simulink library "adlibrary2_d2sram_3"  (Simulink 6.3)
undefined symbols (not defined in the file or in its folder): adlibrary2_zbt32_0, b9ac2330, Bit, Black, blackbox2, blue, Box1, d2sram_config, gcbh, Generation, Inactive, Location, Lower, SRAM, VER_STRING_GOES_HERE, white, Width, xlBlockLoadCallback, ZBT
libraries: xbsIndex_r4 x25, adlibrary2_d2sram_0 x1

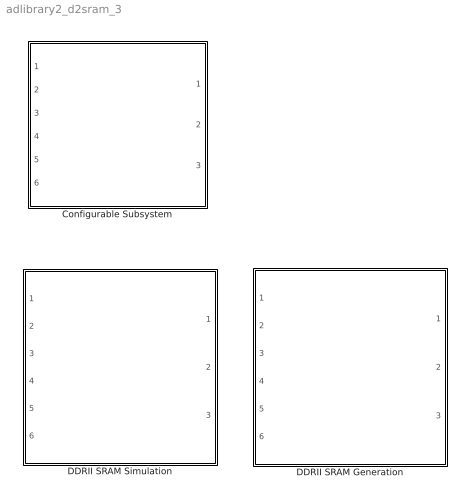
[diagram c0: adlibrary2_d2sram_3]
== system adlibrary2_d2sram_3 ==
  Configurable Subsystem : Subsystem  Tag=configX  BlockChoice=DDRII SRAM Simulation
  DDRII SRAM Generation : Subsystem
  DDRII SRAM Simulation : Subsystem

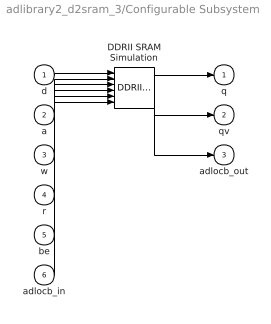
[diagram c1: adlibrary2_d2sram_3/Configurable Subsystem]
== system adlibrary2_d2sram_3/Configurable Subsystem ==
  d : Inport
  a : Inport  Port=2
  w : Inport  Port=3
  r : Inport  Port=4
  be : Inport  Port=5
  adlocb_in : Inport  Port=6
  DDRII SRAM Simulation : adlibrary2_d2sram_0/DDRII SRAM Simulation
  q : Outport
  qv : Outport  Port=2
  adlocb_out : Outport  Port=3
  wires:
  d/1 -> DDRII SRAM Simulation/1
  a/1 -> DDRII SRAM Simulation/2
  w/1 -> DDRII SRAM Simulation/3
  r/1 -> DDRII SRAM Simulation/4
  be/1 -> DDRII SRAM Simulation/5
  adlocb_in/1 -> DDRII SRAM Simulation/6
  DDRII SRAM Simulation/1 -> q/1
  DDRII SRAM Simulation/2 -> qv/1
  DDRII SRAM Simulation/3 -> adlocb_out/1

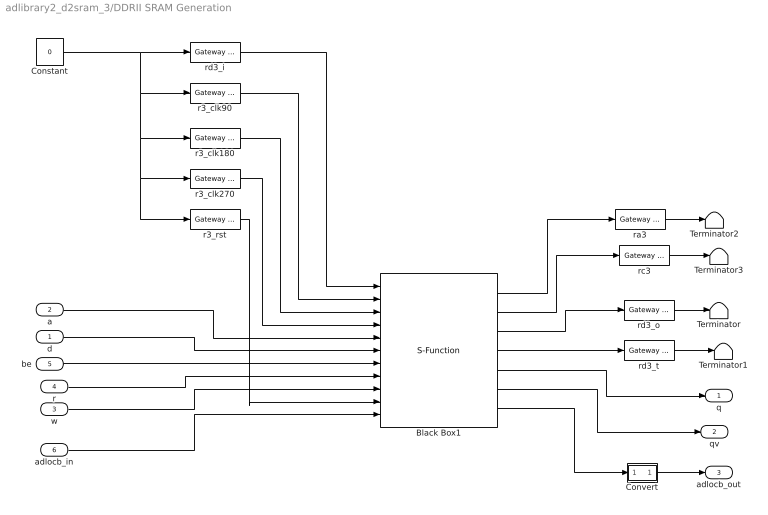
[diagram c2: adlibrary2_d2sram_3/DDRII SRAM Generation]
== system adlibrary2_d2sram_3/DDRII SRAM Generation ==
  d : Inport
  a : Inport  Port=2
  w : Inport  Port=3
  r : Inport  Port=4
  be : Inport  Port=5
  adlocb_in : Inport  Port=6
  Black Box1 : S-Function  AncestorBlock=adlibrary2_zbt32_0/ZBT SRAM 32Bit Generation/Black Box1  LoadFcn=xlBlockLoadCallback(gcbh);  FunctionName=sysgen  Parameters=ptable_  mask(Xilinx Black Box Block){infoedit=Incorporates black box HDL and simulation model into a System Generator design.<P><P>You must supply a Black Box with certain information about the HDL component you would like to bring into System Generator. This information is provided through a Matlab function.<P><P>When "Simulation mode" is set to "Inactive", you will typically want to provide a separate simulation model by using a Simulation 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, init_code=d2sram_config, sim_method=Inactive, sim_method_sgadvanced=, engine_block=, xl_use_area=off, xl_use_area_sgadvanced=, xl_area=[0,0,0,0,0,0,0], block_version=VER_STRING_GOES_HERE, has_advanced_control=0, sggui_pos=20,20,356,367, block_type=blackbox2, sg_icon_stat=130,170,11,7,white,blue,0,b9ac2330, sg_mask_display=fprintf('','COMMENT: begin icon graphics '); patch([0 130 130 0 ],[0 0 170 170 ],[0.77 0.82 0.91]); patch([31 9 39 9 31 65 74 83 120 91 63 43 74 43 63 91 120 83 74 65 31 ],[34 56 86 116 138 138 129 138 138 109 137 117 86 55 35 63 34 34 43 34 34 ],[0.98 0.96 0.92]); plot([0 0 130 130 0 ],[0 170 170 0 0 ]); fprintf('','COMMENT: end icon graphics');  fprintf('','COMMENT: begin icon text '); color('bl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, sg_list_contents=, adlocb_devid=3}
      mask prompts: infoedit ""; init_code "Block configuration m-function"; sim_method "Simulation mode"; engine_block "HDL co-simulator to use  (specify helper block by name)"; xl_use_area "Define FPGA area for resource estimation"; xl_area "FPGA area [slices, FFs, BRAMs, LUTs, IOBs, emb. mults, TBUFs]"; block_version ""; has_advanced_control ""; sggui_pos ""; block_type ""; sg_icon_stat ""; sg_mask_display ""; sg_list_contents ""; adlocb_devid "ADLOCB DEV ID"
      mask help: Incorporates black box HDL and simulation model into a System Generator design. You must supply a Black Box with certain information about the HDL component you would like to bring into System Generator. This information is provided through a Matlab function. When "Simulation mode" is set to "Inactive", you will typically want to provide a separate simulation model by using a Simulation Multiplexer. When "Simulation mode" is set to "External co-simulator", you must include a ModelSim block in the design.
      mask init:
      | xlMungeMaskParams;
      | 
      | mdlPath = xlGetMdlDir(bdroot);
      | 
      | refBlk = get_param(gcb,'referenceBlock');
      | if (isempty(refBlk) | strncmp(refBlk,'xbsIndex',8))
      | srcPath = mdlPath;
      | else
      | srcPath = xlPathToReference;
      | if (isempty(srcPath))
      | srcPath = mdlPath;
      | end
      | end
      | 
      | if (sim_method==3)
      | validEngineBlock = 0;
      | try
      | engineBlock = xlBlockNameRelPath(get_param(gcb,'Parent'),engine_block);
      | catch
      | engineBlock = '//';
      | end
      | try 
      | engineWorkDir = get_param(engineBlock,'dir');
      | validEngineBlock = 1;
      | engine_handle = get_param(engineBlock,'Handle');
      | catch
      | end
      | end
      | 
      | % build black box config function
      | block_config = ['sysgen:black_box_config:' init_code];
      | 
      | serialized_declarations = '{''engine_handle''=>''Double'',''sim_method''=>''Int'',''validEngineBlock''=>''Int'',''engineWorkDir''=>''String'',''engine_block''=>''String'',''init_code''=>''String'',''mdlPath''=>''String'',''srcPath''=>''String'',''block_config''=>''String'',}';
      | ptable_ = xlblockprep(get_param(gcb, 'MaskWSVariables'));
  Constant : Constant  Value=0
  Convert : Subsystem
  Terminator{,1..3} (4 alike) : Terminator
  r3_clk180 : xbsIndex_r4/Gateway In  arith_type=Boolean  n_bits=1  bin_pt=0  period=ad_get_simulink_period  dbl_ovrd=off  timing_constraint=None  locs_specified=off  LOCs={}  block_type=gatewayin
  r3_clk270 : xbsIndex_r4/Gateway In  arith_type=Boolean  n_bits=1  bin_pt=0  period=ad_get_simulink_period  dbl_ovrd=off  timing_constraint=None  locs_specified=off  LOCs={}  block_type=gatewayin
  r3_clk90 : xbsIndex_r4/Gateway In  arith_type=Boolean  n_bits=1  bin_pt=0  period=ad_get_simulink_period  dbl_ovrd=off  timing_constraint=None  locs_specified=off  LOCs={}  block_type=gatewayin
  r3_rst : xbsIndex_r4/Gateway In  arith_type=Boolean  n_bits=1  bin_pt=0  period=ad_get_simulink_period  dbl_ovrd=off  timing_constraint=None  locs_specified=off  LOCs={}  block_type=gatewayin
  ra3 : xbsIndex_r4/Gateway Out  hdl_port=on  timing_constraint=None  locs_specified=off  LOCs={}  block_type=gatewayout
  rc3 : xbsIndex_r4/Gateway Out  hdl_port=on  timing_constraint=None  locs_specified=off  LOCs={}  block_type=gatewayout
  rd3_i : xbsIndex_r4/Gateway In  arith_type=Unsigned  n_bits=32  bin_pt=0  period=ad_get_simulink_period  dbl_ovrd=off  timing_constraint=None  locs_specified=off  LOCs={}  block_type=gatewayin
  rd3_o : xbsIndex_r4/Gateway Out  hdl_port=on  timing_constraint=None  locs_specified=off  LOCs={}  block_type=gatewayout
  rd3_t : xbsIndex_r4/Gateway Out  hdl_port=on  timing_constraint=None  locs_specified=off  LOCs={}  block_type=gatewayout
  q : Outport
  qv : Outport  Port=2
  adlocb_out : Outport  Port=3
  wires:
  rc3/1 -> Terminator3/1
  ra3/1 -> Terminator2/1
  rd3_t/1 -> Terminator1/1
  rd3_o/1 -> Terminator/1
  Constant/1 -> rd3_i/1, r3_rst/1, r3_clk270/1, r3_clk180/1, r3_clk90/1
  be/1 -> Black Box1/7
  d/1 -> Black Box1/6
  a/1 -> Black Box1/5
  w/1 -> Black Box1/9
  r/1 -> Black Box1/8
  Black Box1/4 -> rd3_t/1
  Black Box1/3 -> rd3_o/1
  Black Box1/2 -> rc3/1
  Black Box1/1 -> ra3/1
  Black Box1/5 -> q/1
  r3_rst/1 -> Black Box1/10
  r3_clk270/1 -> Black Box1/4
  r3_clk180/1 -> Black Box1/3
  r3_clk90/1 -> Black Box1/2
  rd3_i/1 -> Black Box1/1
  Black Box1/6 -> qv/1
  Convert/1(out0) -> adlocb_out/1
  adlocb_in/1 -> Black Box1/11
  Black Box1/7 -> Convert/1(in0)

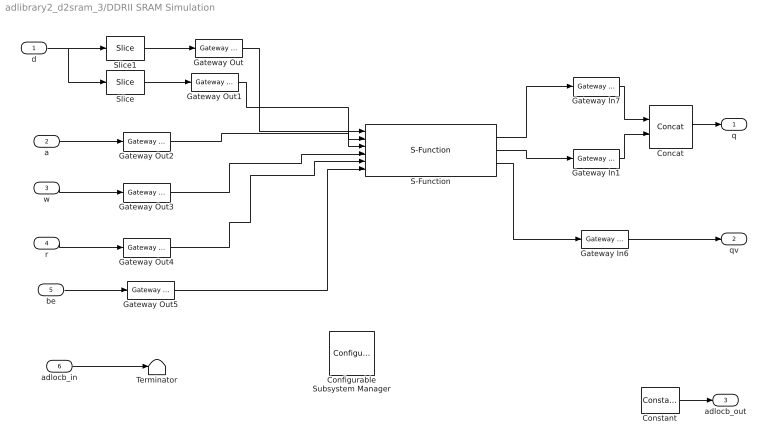
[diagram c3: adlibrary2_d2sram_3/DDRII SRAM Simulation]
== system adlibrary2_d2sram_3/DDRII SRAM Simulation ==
  d : Inport
  a : Inport  Port=2
  w : Inport  Port=3
  r : Inport  Port=4
  be : Inport  Port=5
  adlocb_in : Inport  Port=6
  Concat : xbsIndex_r4/Concat  num_inputs=2  dbl_ovrd=off  block_type=concat
  Configurable Subsystem Manager : xbsIndex_r4/Configurable Subsystem Manager  Tag=xcfgMgr  block_type=configsubsys
  Constant : xbsIndex_r4/Constant  arith_type=Signed (2's comp)  const=0  n_bits=66  bin_pt=0  explicit_period=on  period=ad_get_simulink_period  equ=P=C  opselect=C  inp2=PCIN>>17  opr=+  inp1=P  carry=CIN  dbl_ovrd=off  block_type=constant
  Gateway In1 : xbsIndex_r4/Gateway In  arith_type=Unsigned  n_bits=32  bin_pt=0  period=ad_get_simulink_period  dbl_ovrd=on  timing_constraint=None  locs_specified=off  LOCs={}  block_type=gatewayin
  Gateway In6 : xbsIndex_r4/Gateway In  arith_type=Boolean  n_bits=1  bin_pt=0  period=ad_get_simulink_period  dbl_ovrd=on  timing_constraint=None  locs_specified=off  LOCs={}  block_type=gatewayin
  Gateway In7 : xbsIndex_r4/Gateway In  arith_type=Unsigned  n_bits=32  bin_pt=0  period=ad_get_simulink_period  dbl_ovrd=on  timing_constraint=None  locs_specified=off  LOCs={}  block_type=gatewayin
  Gateway Out{,1..5} (6 alike) : xbsIndex_r4/Gateway Out  hdl_port=off  timing_constraint=None  locs_specified=off  LOCs={}  block_type=gatewayout
  S-Function : S-Function  FunctionName=d2sram  Parameters=3
  Slice : xbsIndex_r4/Slice  nbits=32  boolean_output=off  mode=Lower Bit Location + Width  bit1=0  base1=MSB of Input  bit0=0  base0=LSB of Input  dbl_ovrd=off  block_type=slice
  Slice1 : xbsIndex_r4/Slice  nbits=32  boolean_output=off  mode=Lower Bit Location + Width  bit1=0  base1=MSB of Input  bit0=32  base0=LSB of Input  dbl_ovrd=off  block_type=slice
  Terminator : Terminator
  q : Outport
  qv : Outport  Port=2
  adlocb_out : Outport  Port=3
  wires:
  Concat/1 -> q/1
  Gateway In1/1 -> Concat/2
  Gateway In7/1 -> Concat/1
  d/1 -> Slice/1, Slice1/1
  Slice/1 -> Gateway Out1/1
  Slice1/1 -> Gateway Out/1
  Gateway Out5/1 -> S-Function/6
  be/1 -> Gateway Out5/1
  S-Function/3 -> Gateway In6/1
  Gateway In6/1 -> qv/1
  S-Function/2 -> Gateway In1/1
  Gateway Out4/1 -> S-Function/5
  r/1 -> Gateway Out4/1
  Gateway Out3/1 -> S-Function/4
  Gateway Out2/1 -> S-Function/3
  Gateway Out1/1 -> S-Function/2
  Gateway Out/1 -> S-Function/1
  S-Function/1 -> Gateway In7/1
  w/1 -> Gateway Out3/1
  a/1 -> Gateway Out2/1
  Constant/1 -> adlocb_out/1
  adlocb_in/1 -> Terminator/1

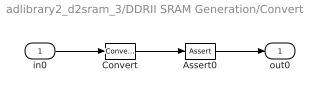
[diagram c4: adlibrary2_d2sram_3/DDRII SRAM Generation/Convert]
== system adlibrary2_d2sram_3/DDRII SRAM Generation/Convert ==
  in0 : Inport
  Assert0 : xbsIndex_r4/Assert  assert_type=off  type_source=Explicitly  arith_type="Signed  (2's comp)"  n_bits=16  bin_pt=14  assert_rate=on  rate_source=Explicitly  period=ad_get_simulink_period  output_port=on  block_type=assert
  Convert : xbsIndex_r4/Convert  arith_type=Unsigned  n_bits=66  bin_pt=0  quantization=Truncate  overflow=Wrap  latency=0  dbl_ovrd=off  pipeline=off  block_type=convert
  out0 : Outport
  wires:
  in0/1 -> Convert/1
  Convert/1 -> Assert0/1
  Assert0/1 -> out0/1
